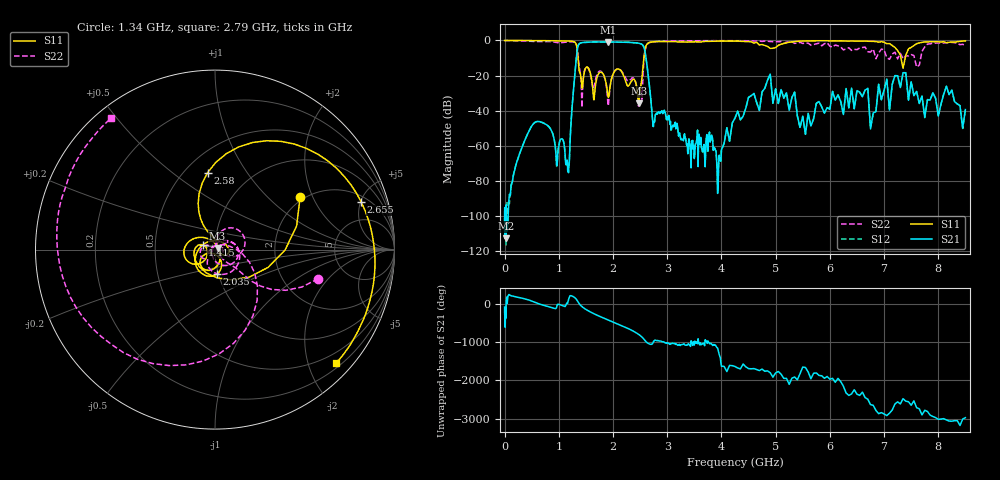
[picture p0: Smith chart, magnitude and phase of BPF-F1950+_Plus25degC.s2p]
! Mini-Circuits
! S2P DATA File Format
! Type: BAND PASS FILTER
! Model: BPF-F1950+
! All S Parameters are in dB deg format
! TEST CONDITIONS: INPUT POWER = 0 dBm @ Temperature = +25deg C
# MHz S dB R 50
!Frequency  S11 dB  S11 DEG  S21 dB  S21 DEG  S12 dB  S12 DEG  S22 dB  S22 DEG
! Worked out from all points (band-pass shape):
!   712 points, 1 MHz to 8.5 GHz, reference 50 ohm
!   highest |S21| = -0.79 dB at 1.915 GHz (marker M1); lowest = -112.8 dB at 21 MHz (marker M2)
!   |S21| within 3 dB of the highest: 1.351 GHz to 2.569 GHz (1.219 GHz wide, 62.2 % of centre)
!   lowest |S11| = -35.9 dB at 2.475 GHz (marker M3), VSWR 1.03, Z = 51.4 + j0.81 ohm
!   |S11| at or under -10 dB: 1.355 GHz to 2.569 GHz (1.215 GHz wide, 61.9 % of centre); 7.311 GHz to 7.39 GHz (79.03 MHz wide, 1.08 % of centre)
!   |S22| runs from -38.2 to 0.0 dB; largest |S21 - S12| = 0.0068
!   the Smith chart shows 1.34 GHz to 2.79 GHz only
!   S11 on the Smith chart (normalised r, x): 1.34 GHz: 1.91, +1.61; 1.415 GHz: 0.87, +0.05; 2.035 GHz: 0.98, -0.27; 2.58 GHz: 0.64, +0.68; 2.655 GHz: 2.54, +5.06; 2.79 GHz: 0.28, -2.50
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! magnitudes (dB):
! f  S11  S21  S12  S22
! 1 MHz  0.0  -102.3  -102.3  -0.1
! 21 MHz  0.0  -112.8  -99.2  0.0
! 600 MHz  -0.1  -46.2  -46.3  -0.7
! 1.18 GHz  -0.3  -75.4  -75.1  -0.8
! 1.34 GHz  -5.1  -5.7  -5.7  -4.5
! 1.415 GHz  -22.6  -1.3  -1.3  -25.8
! 1.42 GHz  -24.2  -1.3  -1.3  -29.8
! 1.775 GHz  -18.1  -0.9  -0.9  -17.6
! 1.915 GHz  -32.5  -0.8  -0.8  -37.1
! 2.035 GHz  -17.2  -0.9  -0.9  -17.3
! 2.475 GHz  -35.9  -1.6  -1.6  -36.5
! 2.58 GHz  -7.3  -4.9  -4.9  -8.7
! 2.655 GHz  -1.3  -21.2  -21.2  -1.5
! 2.79 GHz  -0.7  -42.2  -42.2  -0.6
! 2.835 GHz  -0.6  -40.9  -40.8  -0.5
! 3.8 GHz  -0.5  -57.0  -57.0  -0.1
! 3.95 GHz  -0.4  -69.2  -69.2  -0.1
! 4.3 GHz  -0.4  -40.4  -40.3  -0.2
! 4.95 GHz  -4.5  -35.8  -35.8  -0.7
! 5.7 GHz  -0.2  -44.9  -44.3  -2.3
! 7.1 GHz  -1.8  -39.7  -39.8  -10.7
! 8.5 GHz  -0.2  -39.4  -39.5  -2.8
